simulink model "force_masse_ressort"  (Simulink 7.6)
settings: Solver=ode15s  StartTime=0.0  StopTime=10  MaxStep=0.2  RelTol=1e-3
StopFcn:
  | close all, clc
  | load signaux.mat
  | subplot 211
  | plot(x(1,:),x(2,:))
  | title('Masse-ressort, mouvement rotationnel')
  | grid
  | axis([0 10 -0.2 1.2])
  | subplot 212
  | plotyy(x(1,:),x(3,:),x(1,:),x(4,:))
  | grid
  | xlabel('temps')
libraries: fl_lib x8, nesl_utility x4

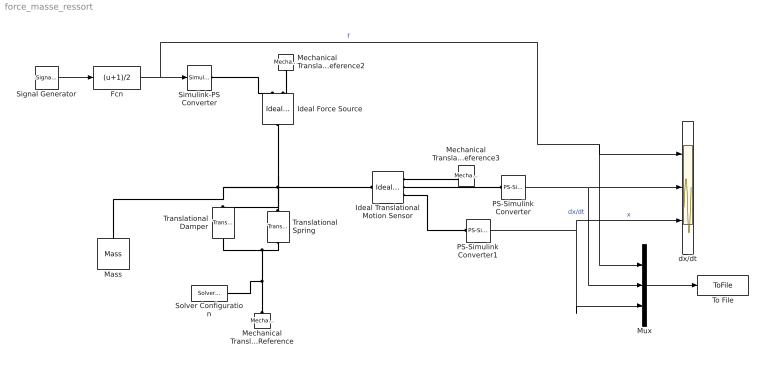
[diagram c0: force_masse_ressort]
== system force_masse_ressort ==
  Fcn : Fcn  Expr=(u+1)/2
  Ideal Force Source : fl_lib/Mechanical/Mechanical Sources/Ideal Force Source  DialogController=NetworkEngine.DynNeDlgSource  SystemSampleTime=-1  v_Log=off  f_Log=off  LocalVarNames=|v|f  LocalVarDescs=|v|f  LocalVarLogging=[0 0]
  Ideal Translational Motion Sensor : fl_lib/Mechanical/Mechanical Sensors/Ideal Translational Motion Sensor  DialogController=NetworkEngine.DynNeDlgSource  SystemSampleTime=-1  offset=0 m  v_Log=off  f_Log=off  x_Log=off  LocalVarNames=|v|f|x  LocalVarDescs=|v|f|x  LocalVarLogging=[0 0 0]
  Mass : fl_lib/Mechanical/Translational Elements/Mass  DialogController=NetworkEngine.DynNeDlgSource  SystemSampleTime=-1  mass=1 kg  initial_velocity=0 m/s  f_Log=off  LocalVarNames=|f  LocalVarDescs=|f  LocalVarLogging=0
  Mechanical Translational Reference : fl_lib/Mechanical/Translational Elements/Mechanical Translational Reference  DialogController=NetworkEngine.DynNeDlgSource  SystemSampleTime=-1  f_Log=off  LocalVarNames=|f  LocalVarDescs=|f  LocalVarLogging=0
  Mechanical Translational Reference2 : fl_lib/Mechanical/Translational Elements/Mechanical Translational Reference  DialogController=NetworkEngine.DynNeDlgSource  SystemSampleTime=-1  f_Log=off  LocalVarNames=|f  LocalVarDescs=|f  LocalVarLogging=0
  Mechanical Translational Reference3 : fl_lib/Mechanical/Translational Elements/Mechanical Translational Reference  DialogController=NetworkEngine.DynNeDlgSource  SystemSampleTime=-1  f_Log=off  LocalVarNames=|f  LocalVarDescs=|f  LocalVarLogging=0
  Mux : Mux  Inputs=3
  PS-Simulink Converter : nesl_utility/PS-Simulink Converter  DialogController=NetworkEngine.DynNeUtilDlgSource  SystemSampleTime=-1  PhysicalDomain=network_engine_domain  LeftPortType=input  RightPortType=output  SubClassName=ps_output  Unit=1  AffineConversion=off
  PS-Simulink Converter1 : nesl_utility/PS-Simulink Converter  DialogController=NetworkEngine.DynNeUtilDlgSource  SystemSampleTime=-1  PhysicalDomain=network_engine_domain  LeftPortType=input  RightPortType=output  SubClassName=ps_output  Unit=1  AffineConversion=off
  Signal Generator : SignalGenerator  WaveForm=square  Frequency=0.2
  Simulink-PS Converter : nesl_utility/Simulink-PS Converter  DialogController=NetworkEngine.DynNeUtilDlgSource  SystemSampleTime=-1  PhysicalDomain=network_engine_domain  LeftPortType=input  RightPortType=output  SubClassName=ps_input  Unit=1  AffineConversion=off  InputFilterTimeConstant=.001  UdotUserProvided=0
  Solver Configuration : nesl_utility/Solver Configuration  DialogController=NetworkEngine.DynNeUtilDlgSource  SystemSampleTime=-1  PhysicalDomain=network_engine_domain  LeftPortType=input  RightPortType=generic  SubClassName=solver  Accelerate=off  Profile=off  ResidualTolerance=1e-9  MaxNonlinIter=12  MaxModeIter=2  DoFixedCost=off  UseLocalSampling=off  DoDC=off  LinearAlgebra=Sparse  LocalSolverSampleTime=.001  LocalSolverChoice=NE_BACKWARD_EULER_ADVANCER  UseLocalSolver=off
  To File : ToFile  Filename=signaux  MatrixName=x
  Translational Damper : fl_lib/Mechanical/Translational Elements/Translational Damper  DialogController=NetworkEngine.DynNeDlgSource  SystemSampleTime=-1  D=100 N/(m/s)  f_Log=off  v_Log=off  LocalVarNames=|f|v  LocalVarDescs=|f|v  LocalVarLogging=[0 0]
  Translational Spring : fl_lib/Mechanical/Translational Elements/Translational Spring  DialogController=NetworkEngine.DynNeDlgSource  SystemSampleTime=-1  spr_rate=1000 N/m  init_def=0 m  f_Log=off  v_Log=off  x_Log=off  LocalVarNames=|f|v|x  LocalVarDescs=|f|v|x  LocalVarLogging=[0 0 0]
  dx/dt : Scope  NumInputPorts=3
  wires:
  PS-Simulink Converter1/1 -> dx/dt/3, Mux/3  "x"
  Signal Generator/1 -> Fcn/1
  Fcn/1 -> Simulink-PS Converter/1, dx/dt/1, Mux/1  "f"
  PS-Simulink Converter/1 -> dx/dt/2, Mux/2  "dx/dt"
  Mux/1 -> To File/1
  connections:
  Ideal Force Source/LConn1 -- Mass/LConn1 -- Translational Damper/LConn1 -- Translational Spring/LConn1 -- Ideal Translational Motion Sensor/LConn1
  Translational Spring/RConn1 -- Translational Damper/RConn1 -- Mechanical Translational Reference/LConn1 -- Solver Configuration/RConn1
  Mechanical Translational Reference2/LConn1 -- Ideal Force Source/RConn2
  Mechanical Translational Reference3/LConn1 -- Ideal Translational Motion Sensor/RConn1
  Simulink-PS Converter/RConn1 -- Ideal Force Source/RConn1
  PS-Simulink Converter/LConn1 -- Ideal Translational Motion Sensor/RConn2
  Ideal Translational Motion Sensor/RConn3 -- PS-Simulink Converter1/LConn1
